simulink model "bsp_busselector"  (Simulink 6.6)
settings: Solver=VariableStepDiscrete  SolverMode=SingleTasking  StartTime=0.0  StopTime=10.0  FixedStep=0.01  RelTol=1e-3

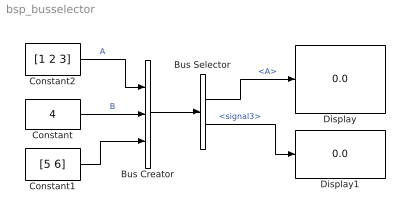
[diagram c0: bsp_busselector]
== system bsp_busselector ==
  Bus Creator : BusCreator  Inputs=3
  Bus Selector : BusSelector  OutputSignals=A,signal3
  Constant : Constant  Value=4
  Constant1 : Constant  Value=[5 6]
  Constant2 : Constant  Value=[1 2 3]
  Display : Display
  Display1 : Display
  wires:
  Constant2/1 -> Bus Creator/1  "A"
  Constant/1 -> Bus Creator/2  "B"
  Bus Creator/1 -> Bus Selector/1
  Bus Selector/2 -> Display1/1  "<signal3>"
  Constant1/1 -> Bus Creator/3
  Bus Selector/1 -> Display/1  "<A>"
